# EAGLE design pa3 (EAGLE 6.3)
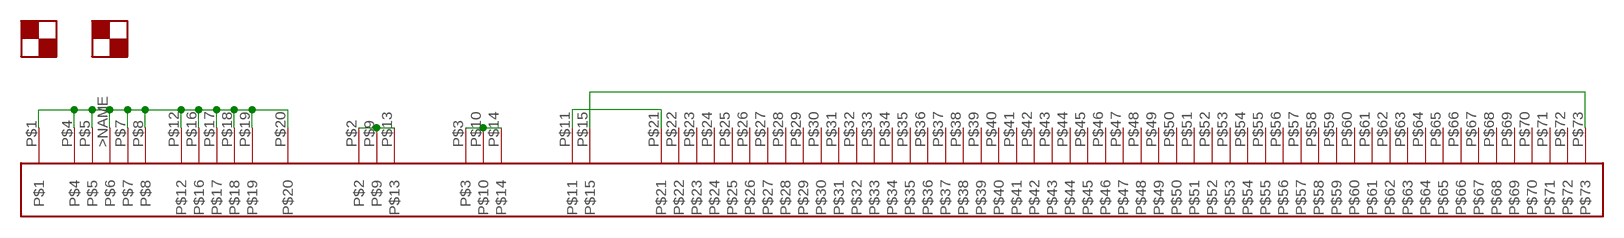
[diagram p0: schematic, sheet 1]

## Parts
PA3  2 x Farnell 1301752  PA3  [PA3]
U$2  AMARK  [AMARK]
U$3  AMARK  [AMARK]

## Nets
N$1: PA3.P$15 PA3.P$73
N$2: PA3.P$2 PA3.P$9 PA3.P$13
N$3: PA3.P$3 PA3.P$10 PA3.P$14
N$4: PA3.>NAME PA3.P$1 PA3.P$4 PA3.P$5 PA3.P$7 PA3.P$8 PA3.P$12 PA3.P$16 PA3.P$17 PA3.P$18 PA3.P$19 PA3.P$20
N$5: PA3.P$11 PA3.P$21
Unconnected: PA3.P$22 PA3.P$23 PA3.P$24 PA3.P$25 PA3.P$26 PA3.P$27 PA3.P$28 PA3.P$29 PA3.P$30 PA3.P$31 PA3.P$32 PA3.P$33 PA3.P$34 PA3.P$35 PA3.P$36 PA3.P$37 PA3.P$38 PA3.P$39 PA3.P$40 PA3.P$41 PA3.P$42 PA3.P$43 PA3.P$44 PA3.P$45 PA3.P$46 PA3.P$47 PA3.P$48 PA3.P$49 PA3.P$50 PA3.P$51 PA3.P$52 PA3.P$53 PA3.P$54 PA3.P$55 PA3.P$56 PA3.P$57 PA3.P$58 PA3.P$59 PA3.P$60 PA3.P$61 PA3.P$62 PA3.P$63 PA3.P$64 PA3.P$65 PA3.P$66 PA3.P$67 PA3.P$68 PA3.P$69 PA3.P$70 PA3.P$71 PA3.P$72

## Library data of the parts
PA3 = FE-I4:PA3
U$2 U$3 = FE-I4:AMARK

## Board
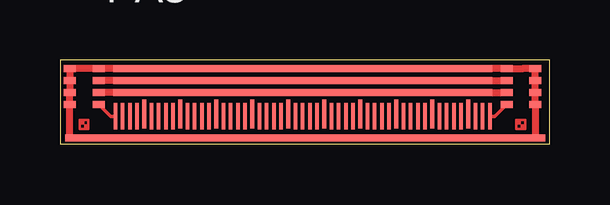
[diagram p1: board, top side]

Size 20.4 x 3.5 mm. Coordinates in mm from the lower left corner, seen from the top.
Outline: 0,0 20.4,0 20.4,3.5 0,3.5 0,0
Copper layers (1*16): Top 0.035mm / dielectric 1.5mm / Bottom 0.035mm
Design rules "default": minimum track width 10mil, minimum drill 24mil, track to track 8mil, track to pad 8mil, pad to pad 8mil, via to via 8mil, smd to smd 8mil, copper to edge 40mil, drill to drill 8mil, minimum pad ring 10mil, minimum via ring 8mil, stop-mask expansion 4mil, vias tented up to drill 0mil, thermal gap 10mil

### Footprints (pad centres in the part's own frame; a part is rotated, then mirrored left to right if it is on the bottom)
PA3 = smd 0.5 x 0.3: >NAME 0.5,-0.3; P$4 0.5,0.7; P$5 0.5,0.2; P$7 0.5,-0.8; P$8 1.7,0.7; P$9 1.7,0.2; P$10 1.7,-0.3; P$11 1.7,-0.8; P$12 18.7,0.7; P$13 18.7,0.2; P$14 18.7,-0.3; P$15 18.7,-0.8; P$16 19.9,0.7; P$17 19.9,0.2; P$18 19.9,-0.3; P$19 19.9,-0.8 | smd 15.8 x 0.3: P$1 10.2,0.7; P$2 10.2,0.2; P$3 10.2,-0.3 | smd 20 x 0.3: P$20 10.3,-2.2 | smd 0.15 x 1.1: P$21 2.4,-1.3; P$22 2.7,-1.3; P$23 3,-1.3; P$24 3.3,-1.3; P$26 3.9,-1.3; P$27 4.2,-1.3; P$28 4.5,-1.3; P$29 4.8,-1.3; P$31 5.4,-1.3; P$32 5.7,-1.3; P$33 6,-1.3; P$34 6.3,-1.3; P$36 6.9,-1.3; P$37 7.2,-1.3; P$38 7.5,-1.3; P$39 7.8,-1.3; P$41 8.4,-1.3; P$42 8.7,-1.3; P$43 9,-1.3; P$44 9.3,-1.3; P$46 9.9,-1.3; P$47 10.2,-1.3; P$48 10.5,-1.3; P$49 10.8,-1.3; P$51 11.4,-1.3; P$52 11.7,-1.3; P$53 12,-1.3; P$54 12.3,-1.3; P$56 12.9,-1.3; P$57 13.2,-1.3; P$58 13.5,-1.3; P$59 13.8,-1.3; P$61 14.4,-1.3; P$62 14.7,-1.3; P$63 15,-1.3; P$64 15.3,-1.3; P$66 15.9,-1.3; P$67 16.2,-1.3; P$68 16.5,-1.3; P$69 16.8,-1.3; P$71 17.4,-1.3; P$72 17.7,-1.3; P$73 18,-1.3 | smd 0.15 x 1.2: P$25 3.6,-1.2; P$30 5.1,-1.2; P$35 6.6,-1.2; P$40 8.1,-1.2; P$45 9.6,-1.2; P$50 11.1,-1.2; P$55 12.6,-1.2; P$60 14.1,-1.2; P$65 15.6,-1.2; P$70 17.1,-1.2

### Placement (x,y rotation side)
PA3  -0.09,2.44 0 top
U$2  1,0.8 0 top
U$3  19.2,0.8 0 top

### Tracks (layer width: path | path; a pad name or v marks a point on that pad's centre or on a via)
N$1
  Top 0.15: PA3.P$73 18.11,1.14 PA3.P$15
N$2
  Top 0.3: PA3.P$9 PA3.P$2 PA3.P$13
N$3
  Top 0.3: PA3.P$10 PA3.P$3 PA3.P$14
N$4
  Top 0.3: PA3.P$1 PA3.P$8 | PA3.P$8 PA3.P$4 PA3.P$5 PA3.>NAME PA3.P$7 0.41,0.24 PA3.P$20 19.81,0.24 PA3.P$19 PA3.P$18 PA3.P$17 PA3.P$16 19.3,3.14 PA3.P$12 PA3.P$8
N$5
  Top 0.15: PA3.P$21 2.11,1.14 PA3.P$11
